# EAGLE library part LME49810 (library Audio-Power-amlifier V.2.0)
LME49810 200V Audio Power Amplifier Driver with Baker Clamp. The LME49810 is a high fidelity audio power amplifier driver designed for demanding consumer and pro-audio applications. Amplifier output power may be scaled by changing the supply voltage and number of power transistors. The LME49810’s minimum output current is 50mA. When using a discrete output stage the LME49810 is capable of delivering in excess of 300 watts into a single-ended 8Ω load.
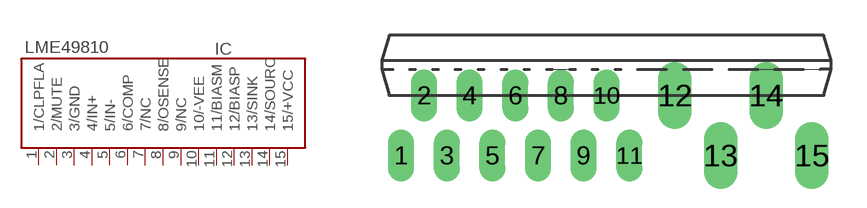
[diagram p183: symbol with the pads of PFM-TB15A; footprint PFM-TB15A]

Designator prefix IC

## LME49810  [PFM-TB15A]
1  1/CLPFLA  out
2  2/MUTE  in
3  3/GND  pwr
4  4/IN+  in
5  5/IN-  in
6  6/COMP
7  7/NC  nc
8  8/OSENSE  out
9  9/NC  nc
10  10/-VEE  pwr
11  11/BIASM
12  12/BIASP
13  13/SINK  out
14  14/SOURC  out
15  15/+VCC  pwr

## Footprint PFM-TB15A (pad centres in mm)
www.ti.com/audio
drill 0.6 long: 1 -8.685,-2.54; 2 -7.72,-0.001; 3 -6.754,-2.54; 4 -5.789,-0.001; 5 -4.824,-2.541; 6 -3.859,-0.001; 7 -2.894,-2.541; 8 -1.929,-0.001; 9 -0.964,-2.541; 10 0.001,-0.001; 11 0.966,-2.541
drill 0.6 pad 1.422 long: 12 2.896,-0.001; 13 4.826,-2.541; 14 6.756,-0.001; 15 8.686,-2.542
